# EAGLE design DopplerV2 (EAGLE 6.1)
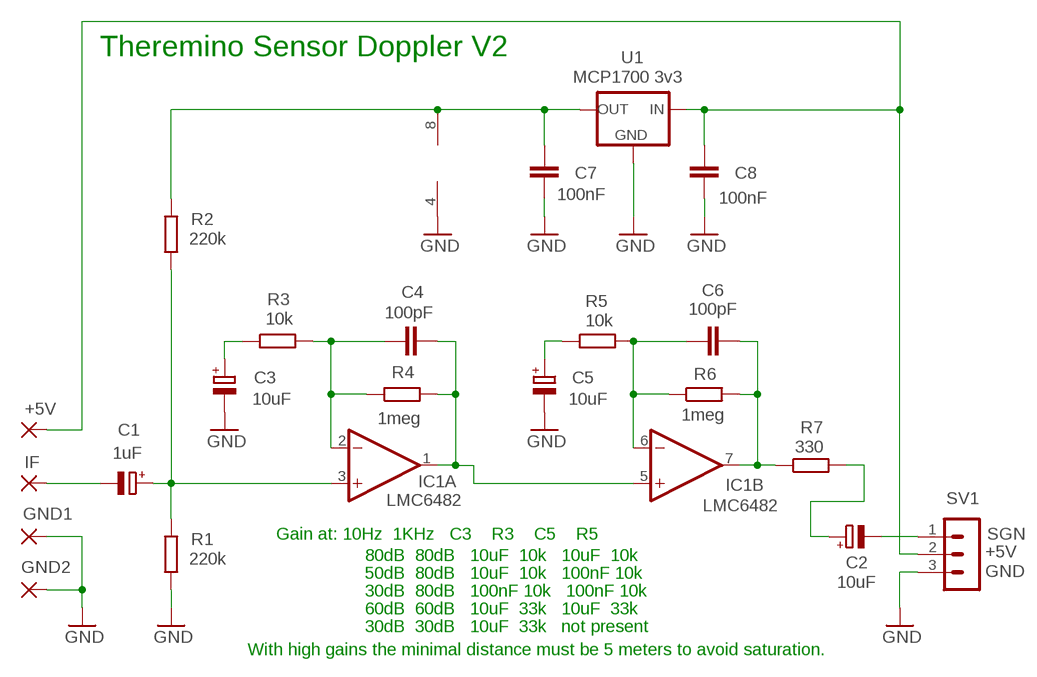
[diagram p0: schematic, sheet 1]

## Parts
+5V  WIREPAD2,54/1,0  [2,54/1,0]
C1  1uF  CPOL-EUE5-4  [E5-4]
C2  10uF  CPOL-EUE2-5B  [E2-5B]
C3  10uF  CPOL-EUE2-5B  [E2-5B]
C4  100pF  C-EU025-024X044  [C025-024X044]
C5  10uF  CPOL-EUE2-5B  [E2-5B]
C6  100pF  C-EU025-024X044  [C025-024X044]
C7  100nF  C-EU050-024X044  [C050-024X044]
C8  100nF  C-EU025-024X044  [C025-024X044]
GND1  WIREPAD2,54/1,0  [2,54/1,0]
GND2  WIREPAD2,54/1,0  [2,54/1,0]
IC1  LMC6482  TL072P  [DIL08]
IF  WIREPAD2,54/1,0  [2,54/1,0]
R1  220k  R-EU_0204/7  [0204/7]
R2  220k  R-EU_0204/7  [0204/7]
R3  10k  R-EU_0204/7  [0204/7]
R4  1meg  R-EU_0204/7  [0204/7]
R5  10k  R-EU_0204/7  [0204/7]
R6  1meg  R-EU_0204/7  [0204/7]
R7  330  R-EU_0204/7  [0204/7]
SV1  MA03-1W  [MA03-1W]
U1  MCP1700 3v3  MCP1700L1  [TO92L1]

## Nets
GND: C3.- C5.- C7.2 C8.2 GND1.1(P) GND2.1(P) IC1.4(P:V-) R1.1 SV1.3 U1.3(GND)
N$1: C4.1 IC1.2(A:-IN) R3.2 R4.1
N$2: C6.1 IC1.6(B:-IN) R5.2 R6.1
N$4: C3.+ R3.1
N$5: C6.2 IC1.7(B:OUT) R6.2 R7.1
N$6: C4.2 IC1.1(A:OUT) IC1.5(B:+IN) R4.2
N$7: C2.- SV1.1
N$8: +5V.1(P) C8.1 SV1.2 U1.2(IN)
N$9: C1.+ IC1.3(A:+IN) R1.2 R2.1
N$10: C7.1 IC1.8(P:V+) R2.2 U1.1(OUT)
N$11: C1.- IF.1(P)
N$12: C2.+ R7.2
N$13: C5.+ R5.1

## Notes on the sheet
- Theremino Sensor Doppler V2
- Gain at: 10Hz  1KHz   C3    R3    C5    R5 | SGN
- 80dB  80dB   10uF  10k   10uF  10k | +5V
- 50dB  80dB   10uF  10k   100nF 10k | GND
- 30dB  80dB   100nF 10k   100nF 10k
- 60dB  60dB   10uF  33k   10uF  33k
- 30dB  30dB   10uF  33k   not present
- With high gains the minimal distance must be 5 meters to avoid saturation.

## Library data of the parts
+5V GND1 GND2 IF = wirepad:WIREPAD: Wire PAD connect wire on PCB
C1-C3 C5 = 00-LIVIO:CPOL-EU: POLARIZED CAPACITOR, European symbol
C4 C6-C8 = 00-LIVIO:C-EU: CAPACITOR, European symbol
IC1 = linear:TL072: OP AMP
R1-R7 = 00-LIVIO:R-EU_: RESISTOR, European symbol
SV1 = 03-con-lstb-M:MA03-1W
U1 = 00-LIVIO:MCP1700: Linear regulator Quescient courrent 1.8uA Input 2.3v to 6v Output 1.2v 1.8v 2.5v 3.0v 3.3v 5.0v

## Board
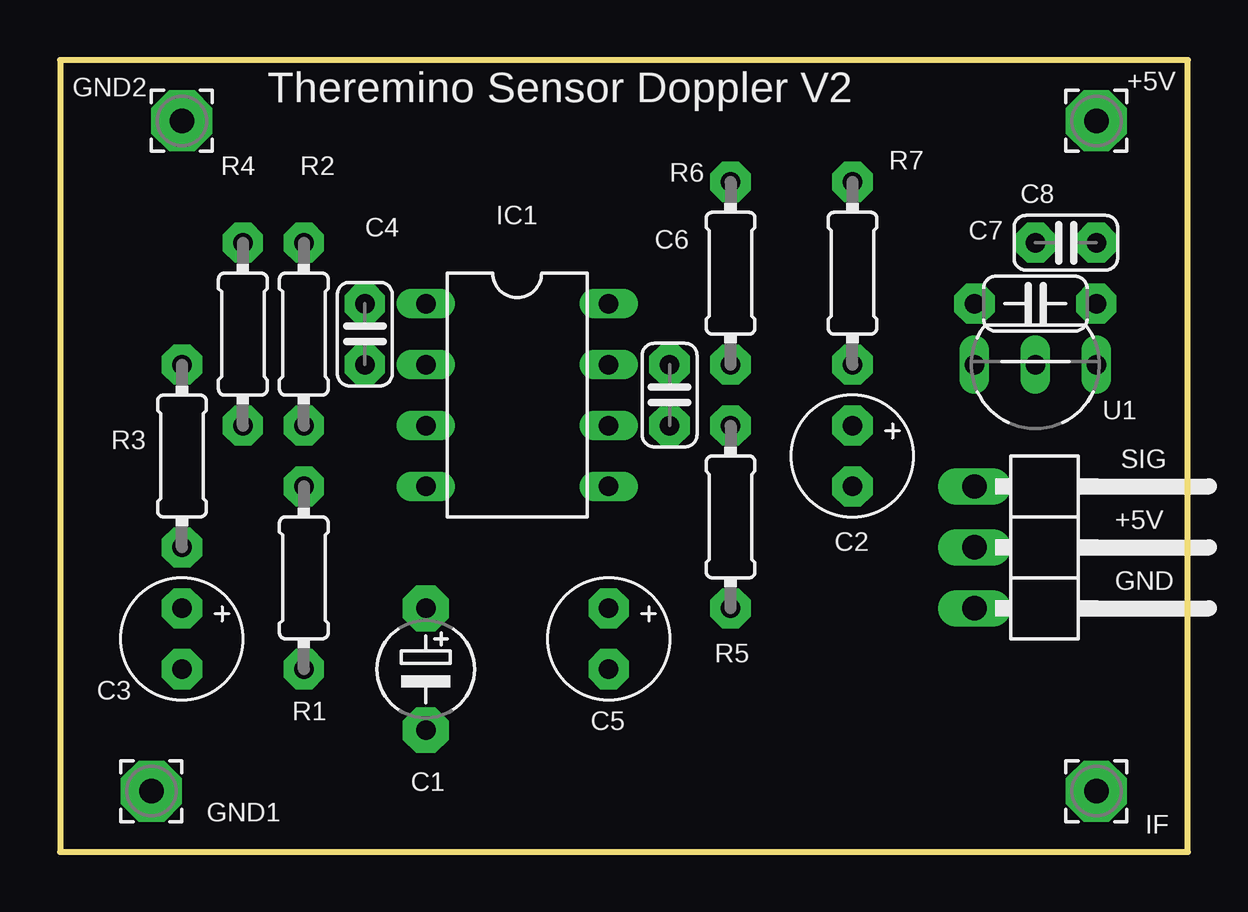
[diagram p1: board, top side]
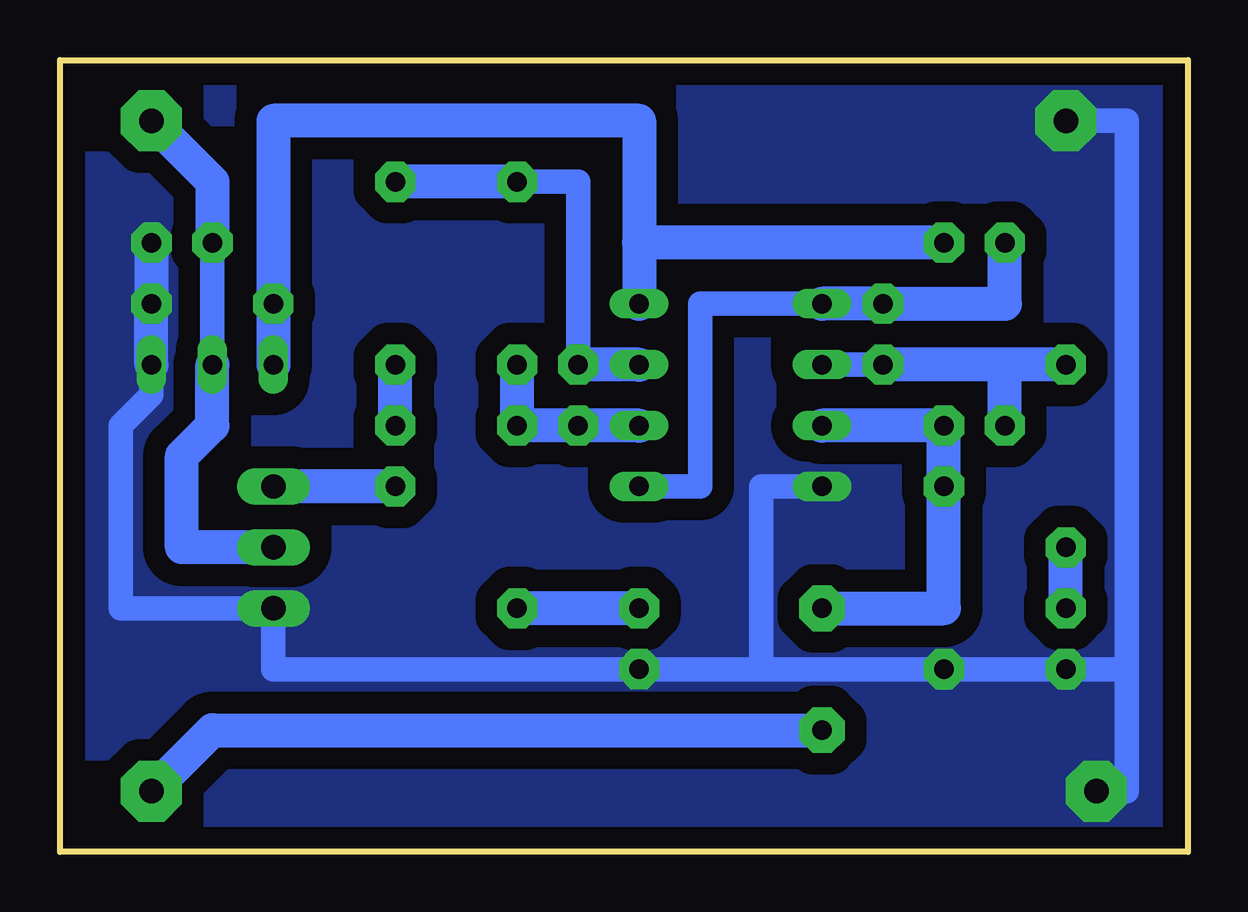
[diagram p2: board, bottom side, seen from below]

Size 46.99 x 33.02 mm. Coordinates in mm from the lower left corner, seen from the top.
Outline: 0,0 46.99,0 46.99,33.02 0,33.02 0,0
Copper layers (1*16): Top 0.035mm / dielectric 1.5mm / Bottom 0.035mm
Design rules: minimum track width 10mil, minimum drill 31mil, track to track 31mil, track to pad 31mil, pad to pad 31mil, via to via 31mil, smd to smd 31mil, copper to edge 31mil, drill to drill 8mil, minimum pad ring 5mil, minimum via ring 8mil, stop-mask expansion 4mil, vias tented up to drill 0mil, thermal gap 47mil

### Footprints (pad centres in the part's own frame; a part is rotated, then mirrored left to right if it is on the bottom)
2,54/1,0 = drill 1.016 pad 2.54 octagon: 1 0,0
E5-4 = drill 0.813 pad 1.905 octagon: + -2.54,0; - 2.54,0
E2-5B = drill 0.813 pad 1.676 octagon: + -1.27,0; - 1.27,0
C025-024X044 = drill 0.813 pad 1.676 octagon: 1 -1.27,0; 2 1.27,0
C050-024X044 = drill 0.813 pad 1.676 octagon: 1 -2.54,0; 2 2.54,0
DIL08 = drill 0.813 long: 1 -3.81,-3.81; 2 -1.27,-3.81; 3 1.27,-3.81; 4 3.81,-3.81; 5 3.81,3.81; 6 1.27,3.81; 7 -1.27,3.81; 8 -3.81,3.81
0204/7 = drill 0.813 pad 1.676 octagon: 1 -3.81,0; 2 3.81,0
MA03-1W = drill 1.016 long: 1 -2.54,0; 2 0,0; 3 2.54,0
TO92L1 = drill 0.813 long: 1 2.54,0; 2 0,0; 3 -2.54,0

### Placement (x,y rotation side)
+5V  43.18,30.48 0 top
C1  15.24,7.62 270 top
C2  33.02,16.51 270 top
C3  5.08,8.89 270 top
C4  12.7,21.59 90 top
C5  22.86,8.89 270 top
C6  25.4,19.05 90 top
C7  40.64,22.86 0 top
C8  41.91,25.4 0 top
GND1  3.81,2.54 0 top
GND2  5.08,30.48 0 top
IC1  19.05,19.05 270 top
IF  43.18,2.54 0 top
R1  10.16,11.43 90 top
R2  10.16,21.59 90 top
R3  5.08,16.51 90 top
R4  7.62,21.59 90 top
R5  27.94,13.97 90 top
R6  27.94,24.13 90 top
R7  33.02,24.13 270 top
SV1  38.1,12.7 270 top
U1  40.64,20.32 180 top

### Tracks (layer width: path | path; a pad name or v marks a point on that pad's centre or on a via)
GND
  Bottom 1.016: 17.78,7.62 20.32,7.62 C5.- 38.1,7.62 SV1.3 44.45,10.16 44.45,17.78 43.18,19.05 U1.3 | 17.78,7.62 17.78,15.24 IC1.4 | 17.78,7.62 R1.1 C3.- 2.54,7.62 | GND1.1 2.54,2.54 2.54,7.62 | 2.54,7.62 2.54,30.48 GND2.1
  Bottom 1.422: U1.3 C7.2 C8.2
  pour Bottom (isolate 0.9, rank 6, no thermals): -1,-1 47.99,-1 47.99,34.02 -1,34.02
N$1
  Bottom 1.016: C4.1 IC1.2
  Bottom 1.422: R3.2 7.62,20.32 | R4.1 7.62,20.32 | 7.62,20.32 C4.1
N$2
  Bottom 1.422: IC1.6 C6.1 R5.2 R6.1
N$4
  Bottom 1.422: C3.+ R3.1
N$5
  Bottom 1.016: C6.2 25.4,27.94 R6.2
  Bottom 1.422: IC1.7 C6.2 | R6.2 R7.1
N$6
  Bottom 1.016: IC1.5 20.32,15.24 20.32,22.86 IC1.1
  Bottom 1.422: IC1.1 C4.2 7.62,22.86 R4.2
N$7
  Bottom 1.422: C2.- SV1.1
N$8
  Bottom 1.016: U1.2 C8.1
  Bottom 1.422: SV1.2 41.91,12.7 41.91,16.51 40.64,17.78 U1.2 | +5V.1 40.64,27.94 C8.1
N$9
  Bottom 1.422: IC1.3 R2.1 R1.2 10.16,10.16 C1.+
N$10
  Bottom 1.422: R2.2 22.86,25.4 | U1.1 C7.1 38.1,30.48 22.86,30.48 22.86,25.4 | 22.86,25.4 IC1.8
N$11
  Bottom 1.422: IF.1 40.64,5.08 C1.-
N$12
  Bottom 1.422: C2.+ R7.2
N$13
  Bottom 1.422: C5.+ R5.1

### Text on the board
tNames: Theremino Sensor Doppler V2 | SIG | +5V | GND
